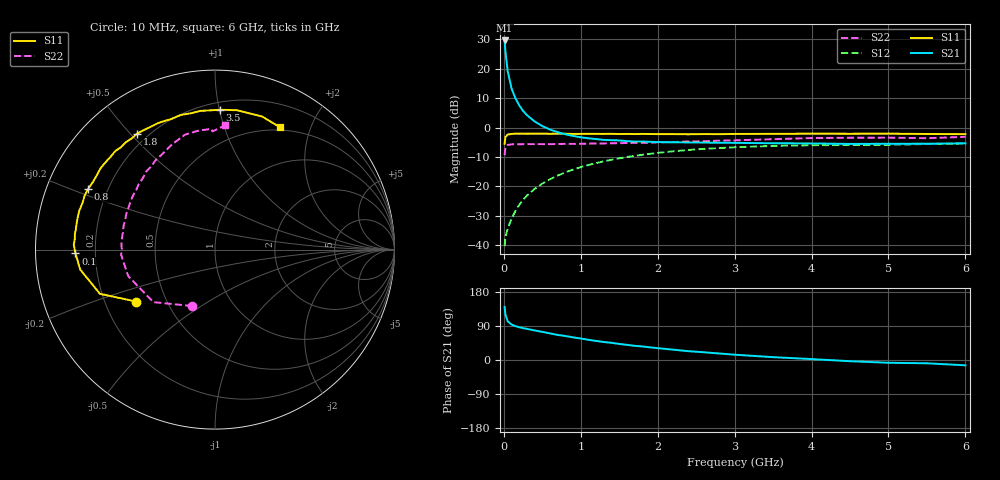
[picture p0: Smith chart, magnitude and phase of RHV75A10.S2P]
! SIEMENS Small Signal Semiconductors
! BFR106
! Si NPN RF Bipolar Junction Transistor in SOT23
! VCE = 0.75 V  IC = 100 mA
! Common Emitter S-Parameters:  August  1996
# GHz  S  MA  R  50
!  f  S11  S21  S12  S22
! GHz  MAG  ANG  MAG  ANG  MAG  ANG  MAG  ANG
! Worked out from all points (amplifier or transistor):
!   36 points, 10 MHz to 6 GHz, reference 50 ohm
!   highest |S21| = 29.6 dB at 10 MHz (marker M1)
!   |S21| within 3 dB of that: start of sweep to 18.49 MHz
!   unconditionally stable (mu >= 1): start of sweep to 18.83 MHz; 23.92 MHz to end of sweep
!   at 250 MHz: K = 1.68, MAG = 10.3 dB, |S12| = -24.6 dB
!   at 1.4 GHz: K = 1.30, MAG = 0.0 dB, |S12| = -11.0 dB
!   at 6 GHz: K = 1.04, MAG = -1.2 dB, |S12| = -5.4 dB
!   S11 on the Smith chart (normalised r, x): 10 MHz: 0.33, -0.27; 100 MHz: 0.13, -0.01; 800 MHz: 0.13, +0.22; 1.8 GHz: 0.16, +0.52; 3.5 GHz: 0.25, +1.00; 6 GHz: 0.46, +1.56
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0.01  0.5271 -146.7  30.23 139.8  0.0096 49.9  0.3391 -112.0
0.02  0.6867 -159.0  20.13 120.4  0.0137 43.7  0.4515 -139.6
0.05  0.7586 -171.5  9.089 102.2  0.019 47.5  0.5056 -163.0
0.1  0.7776 -178.4  4.645 93.6  0.0281 58.1  0.5167 -173.5
0.15  0.7874 178.0  3.142 89.5  0.0379 64.5  0.5241 -177.0
0.2  0.7834 175.8  2.384 86.4  0.0484 67.5  0.5183 -179.8
0.25  0.7854 173.4  1.918 84.0  0.0589 69.0  0.5217 177.9
0.3  0.7836 171.7  1.625 82.2  0.0696 70.1  0.5222 176.6
0.4  0.7853 167.9  1.268 78.0  0.0903 70.1  0.5224 173.9
0.5  0.7869 164.3  1.059 74.2  0.1112 69.5  0.522 171.2
0.6  0.7826 160.6  0.922 70.1  0.132 68.0  0.5212 169.1
0.8  0.7838 154.5  0.766 63.3  0.1726 64.6  0.5269 164.7
1.1  0.7824 144.4  0.656 53.3  0.2304 58.8  0.5326 158.4
1.3  0.7782 138.0  0.616 47.5  0.2661 54.4  0.5361 153.8
1.8  0.7783 123.9  0.578 35.7  0.3439 44.1  0.5485 143.6
2.2  0.773 113.9  0.56 27.3  0.3942 36.0  0.5655 135.4
2.6  0.7739 104.2  0.554 20.4  0.433 28.4  0.5838 127.5
3.5  0.7797 87.9  0.54 7.5  0.4864 13.7  0.6331 112.2
4.5  0.7832 75.2  0.526 -3.2  0.5046 0.7  0.6695 97.7
5  0.7866 70.5  0.529 -7.3  0.5084 -4.2  0.6726 91.7
5.5  0.7759 65.7  0.53 -8.7  0.5235 -6.7  0.6583 91.2
6  0.7719 62.1  0.538 -14.0  0.5364 -12.5  0.6944 85.5
